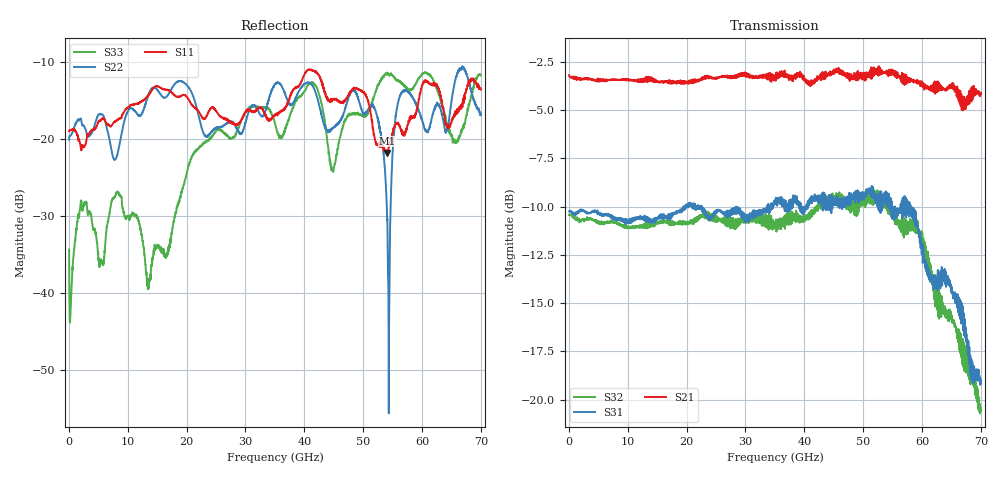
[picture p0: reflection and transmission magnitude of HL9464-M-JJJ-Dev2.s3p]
! 9/8/2020 12:46:25 PM
! H:\PRODUCTION_DATA\TEMP_S3P.S3P
! CHANNEL.1
! TR.MEASUREMENT
! CORRECTED.DATA
# GHZ S RI R 50.0
! FREQ.GHZ  S11RE  S11IM  S12RE  S12IM  S13RE  S13IM
!  S21RE  S21IM  S22RE  S22IM  S23RE  S23IM
!  S31RE  S31IM  S32RE  S32IM  S33RE  S33IM
!; PortSelection: Port_123
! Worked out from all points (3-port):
!   2000 points, 35 MHz to 70 GHz, reference 50 ohm
!   strongest paths, dB at 35 MHz, 17.54 GHz, 35.03 GHz, 52.53 GHz, 70 GHz:
!     S21: -3.2, -3.6, -3.3, -3.2, -4.1
!     S31: -10.2, -10.3, -9.8, -9.5, -19.2
!     S32: -10.4, -10.8, -10.9, -9.3, -20.6
!   lowest |S11| = -21.9 dB at 54.08 GHz (marker M1), VSWR 1.18, Z = 46.4 + j6.92 ohm
!   |S11| at or under -10 dB: start of sweep to end of sweep
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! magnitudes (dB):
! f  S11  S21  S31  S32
! 35 MHz  -19.0  -3.2  -10.2  -10.4
! 2.275 GHz  -20.8  -3.4  -10.2  -10.7
! 13.58 GHz  -14.3  -3.3  -10.7  -10.9
! 21.35 GHz  -16.0  -3.5  -10.1  -10.7
! 35.03 GHz  -16.9  -3.3  -9.8  -10.9
! 51.8 GHz  -19.5  -3.1  -9.2  -9.9
! 54.08 GHz  -21.9  -3.1  -10.0  -9.8
! 56.52 GHz  -18.9  -3.6  -9.8  -10.9
! 65.69 GHz  -16.8  -4.0  -14.6  -16.2
! 70 GHz  -13.6  -4.1  -19.2  -20.6
